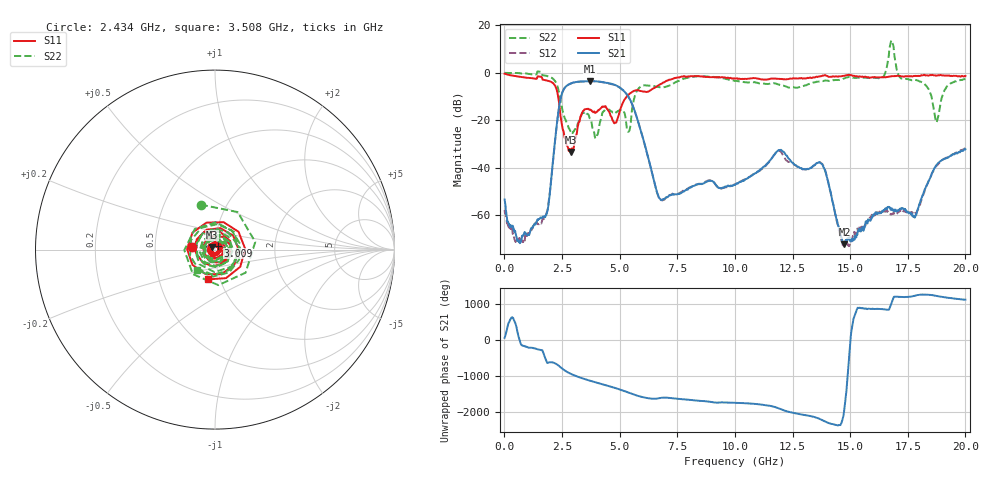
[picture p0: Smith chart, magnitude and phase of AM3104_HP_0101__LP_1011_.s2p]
!Created with skrf (http://scikit-rf.org).
# Hz S RI R 50.0
!freq ReS11 ImS11 ReS21 ImS21 ReS12 ImS12 ReS22 ImS22
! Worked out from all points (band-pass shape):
!   1601 points, 10 MHz to 20 GHz, reference 50 ohm
!   highest |S21| = -3.50 dB at 3.696 GHz (marker M1); lowest = -72.2 dB at 14.75 GHz (marker M2)
!   |S21| within 3 dB of the highest: 2.607 GHz to 5.043 GHz (2.436 GHz wide, 63.7 % of centre)
!   lowest |S11| = -33.4 dB at 2.871 GHz (marker M3), VSWR 1.04, Z = 48.4 + j1.39 ohm
!   |S11| at or under -10 dB: 2.332 GHz to 5.306 GHz (2.973 GHz wide, 77.9 % of centre)
!   |S22| runs from -27.7 to 13.6 dB; largest |S21 - S12| = 0.055
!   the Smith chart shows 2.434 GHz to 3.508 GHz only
!   S11 on the Smith chart (normalised r, x): 2.434 GHz: 0.78, +0.02; 3.009 GHz: 1.03, +0.04; 3.508 GHz: 0.88, -0.30
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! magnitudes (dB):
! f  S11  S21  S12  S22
! 10 MHz  -0.4  -53.4  -57.8  0.0
! 647.2 MHz  -1.7  -71.4  -69.6  -0.2
! 1.784 GHz  -3.1  -60.5  -60.3  -1.2
! 2.434 GHz  -18.0  -11.2  -11.2  -11.6
! 2.871 GHz  -33.4  -4.5  -4.6  -24.7
! 3.009 GHz  -31.5  -4.1  -4.1  -24.7
! 3.346 GHz  -17.6  -3.7  -3.7  -17.6
! 3.508 GHz  -15.4  -3.6  -3.7  -16.5
! 3.696 GHz  -15.6  -3.5  -3.6  -19.1
! 4.808 GHz  -21.1  -5.1  -5.2  -16.9
! 5.395 GHz  -9.2  -10.3  -10.3  -24.8
! 5.807 GHz  -7.4  -20.7  -20.7  -6.8
! 6.682 GHz  -5.3  -52.0  -52.2  -6.0
! 10.01 GHz  -2.5  -47.3  -47.0  -3.4
! 11.93 GHz  -2.5  -32.5  -32.8  -5.0
! 13.34 GHz  -2.1  -39.8  -39.8  -4.3
! 13.87 GHz  -1.1  -40.1  -39.7  -3.3
! 14.75 GHz  -1.2  -72.2  -72.7  -2.3
! 16.68 GHz  -1.6  -56.7  -59.2  7.2
! 17.8 GHz  -1.4  -61.1  -59.3  -3.0
! 18.75 GHz  -1.2  -38.8  -39.2  -20.8
! 20 GHz  -1.4  -32.3  -31.9  -2.6
